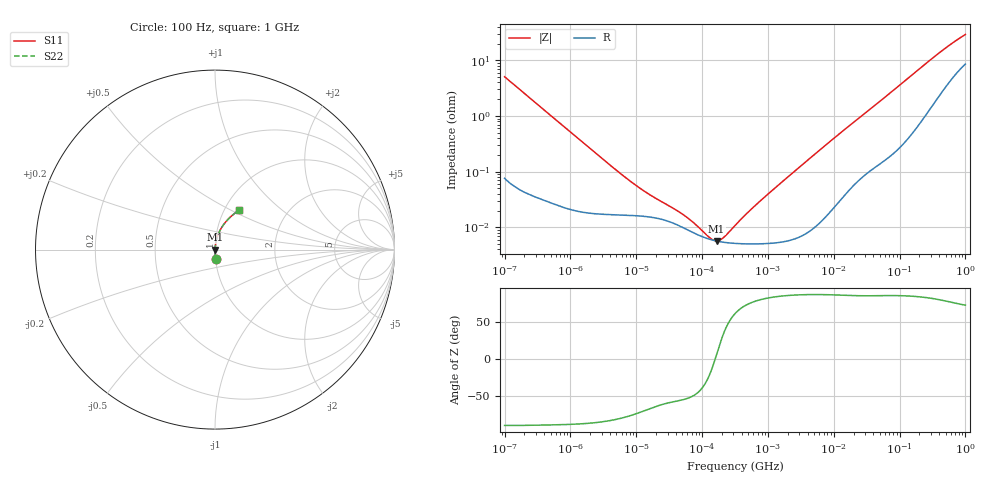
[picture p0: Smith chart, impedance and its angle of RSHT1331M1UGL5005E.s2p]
! RSHT1331M1UGL5005E  S-PARAMETER MODEL  (General Type)
! Model Generated by ELNA Corporation (http://www.ty-top.com)
! Version 1.0
! ELNA Control No.201201
! Copyright (c) 2020 ELNA CO.,LTD. All Rights Reserved.
! Products Name : CONDUCTIVE POLYMER HYBRID ALUMINUM ELECTROLYTIC CAPACITORS
! Characteristics :
!  Capacitance  :  330uF  ,  Rated voltage  :  50V
!  Operating Temp. Range  :  -55 to +105 degC  ,  Endurance  :  10000hr at 105 degC
!  Dimension D  :  12.5mm  ,  Dimension L  :  13.5mm
! Frequency Range : 100Hz - 1GHz
! External Node Assignments :
!  1  o---| |---o  2
# MHz S RI R 50
!Freq[MHz].  S11 Real  S11 Imag  S21 Real  S21 Imag  S12 Real  S12 Imag  S22 Real  S22 Imag
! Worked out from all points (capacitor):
!   401 points, 100 Hz to 1 GHz, reference 50 ohm
!   read as one part in series: C = 314 uF near 108 Hz
!   lowest |Z| = 5.71 mohm at 166 kHz (marker M1)
!   series resonance near 157.6 kHz, so ESL is about 3.3 nH
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0.0001  0.00332 -0.0505  0.9967 0.0505  0.9967 0.0505  0.00332 -0.0505
0.000113  0.00268 -0.0448  0.9973 0.0448  0.9973 0.0448  0.00268 -0.0448
0.000285  0.000673 -0.0178  0.9993 0.0178  0.9993 0.0178  0.000673 -0.0178
0.001488  0.0002 -0.00347  0.9998 0.00347  0.9998 0.00347  0.0002 -0.00347
0.007762  0.000164 -0.000682  0.9998 0.000682  0.9998 0.000682  0.000164 -0.000682
0.013107  0.000158 -0.000421  0.9998 0.000421  0.9998 0.000421  0.000158 -0.000421
0.022131  0.000143 -0.000272  0.9999 0.000272  0.9999 0.000272  0.000143 -0.000272
0.047588  0.000103 -0.000148  0.9999 0.000148  0.9999 0.000148  0.000103 -0.000148
0.087096  7.29e-05 -7.17e-05  0.9999 7.17e-05  0.9999 7.17e-05  7.29e-05 -7.17e-05
0.098288  6.86e-05 -5.69e-05  0.9999 5.69e-05  0.9999 5.69e-05  6.86e-05 -5.69e-05
0.165959  5.67e-05 6.38e-06  0.9999 -6.38e-06  0.9999 -6.38e-06  5.67e-05 6.38e-06
0.280221  5.2e-05 7.61e-05  0.9999 -7.61e-05  0.9999 -7.61e-05  5.2e-05 7.61e-05
0.316228  5.14e-05 9.46e-05  0.9999 -9.46e-05  0.9999 -9.46e-05  5.14e-05 9.46e-05
0.492606  5.04e-05 0.000177  0.9999 -0.000177  0.9999 -0.000177  5.04e-05 0.000177
0.798914  5.07e-05 0.000308  0.9999 -0.000308  0.9999 -0.000308  5.07e-05 0.000308
4.704354  9.52e-05 0.00188  0.9999 -0.00188  0.9999 -0.00188  9.52e-05 0.00188
13.4122  0.000362 0.00524  0.9996 -0.00524  0.9996 -0.00524  0.000362 0.00524
69.9842  0.00247 0.0251  0.9975 -0.0251  0.9975 -0.0251  0.00247 0.0251
169.8244  0.009 0.0589  0.991 -0.0589  0.991 -0.0589  0.009 0.0589
380.1894  0.0358 0.1211  0.9642 -0.1211  0.9642 -0.1211  0.0358 0.1211
641.9482  0.0799 0.1759  0.9201 -0.1759  0.9201 -0.1759  0.0799 0.1759
1000  0.1358 0.2219  0.8642 -0.2219  0.8642 -0.2219  0.1358 0.2219
